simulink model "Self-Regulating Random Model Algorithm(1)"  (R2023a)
settings: Solver=VariableStepAuto  StartTime=0.0  StopTime=20  RelTol=1e-3
libraries: simulink x63, spspowerguiLib x1
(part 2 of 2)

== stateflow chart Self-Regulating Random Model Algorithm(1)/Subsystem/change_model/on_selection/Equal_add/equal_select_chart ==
  state select_num=equal_select(x) [function]
    (default) -> (junction 31)
    (junction 29) -> (junction 65) : {x=x-1}
    (junction 65) -> (junction 118) : [x==0]
    (junction 31) -> (junction 29) : [oo1==1]
    (junction 65) -> (junction 137)
    (junction 118) -> (junction 93) : {select_num=1}
    (junction 31) -> (junction 137)
    (junction 88) -> (junction 91) : {x=x-1}
    (junction 91) -> (junction 89) : [x==0]
    (junction 137) -> (junction 88) : [oo2==1]
    (junction 91) -> (junction 119)
    (junction 89) -> (junction 34) : {select_num=2}
    (junction 137) -> (junction 119)
    (junction 138) -> (junction 142) : {x=x-1}
    (junction 142) -> (junction 143) : [x==0]
    (junction 119) -> (junction 138) : [oo3==1]
    (junction 142) -> (junction 154)
    (junction 143) -> (junction 104) : {select_num=3}
    (junction 119) -> (junction 154)
    (junction 149) -> (junction 153) : {x=x-1}
    (junction 153) -> (junction 155) : [x==0]
    (junction 154) -> (junction 149) : [oo4==1]
    (junction 153) -> (junction 134)
    (junction 155) -> (junction 99) : {select_num=4}
    (junction 154) -> (junction 134)
    (junction 132) -> (junction 131) : {x=x-1}
    (junction 131) -> (junction 128) : [x==0]
    (junction 134) -> (junction 132) : [oo5==1]
    (junction 131) -> (junction 62)
    (junction 128) -> (junction 157) : {select_num=5}
    (junction 134) -> (junction 62)
    (junction 63) -> (junction 61) : {x=x-1}
    (junction 61) -> (junction 59) : [x==0]
    (junction 62) -> (junction 63) : [oo6==1]
    (junction 61) -> (junction 48)
    (junction 59) -> (junction 45) : {select_num=6}
    (junction 62) -> (junction 48)
    (junction 47) -> (junction 46) : {x=x-1}
    (junction 46) -> (junction 49) : [x==0]
    (junction 48) -> (junction 47) : [oo7==1]
    (junction 46) -> (junction 43)
    (junction 49) -> (junction 44) : {select_num=7}
    (junction 48) -> (junction 43)
    (junction 43) -> (junction 35) : [oo8==1]
    (junction 35) -> (junction 41) : {x=x-1}
    (junction 41) -> (junction 39) : [x==0]
    (junction 41) -> (junction 112)
    (junction 43) -> (junction 112)
    (junction 39) -> (junction 148) : {select_num=8}
    (junction 112) -> (junction 111) : [oo9==1]
    (junction 111) -> (junction 110) : {x=x-1}
    (junction 110) -> (junction 107) : [x==0]
    (junction 110) -> (junction 70)
    (junction 112) -> (junction 70)
    (junction 107) -> (junction 95) : {select_num=9}
    (junction 70) -> (junction 69) : [oo10==1]
    (junction 69) -> (junction 67) : {x=x-1}
    (junction 67) -> (junction 66) : [x==0]
    (junction 67) -> (junction 82)
    (junction 70) -> (junction 82)
    (junction 66) -> (junction 122) : {select_num=10}
    (junction 82) -> (junction 86) : [oo11==1]
    (junction 86) -> (junction 79) : {x=x-1}
    (junction 79) -> (junction 84) : [x==0]
    (junction 79) -> (junction 145)
    (junction 82) -> (junction 145)
    (junction 84) -> (junction 96) : {select_num=11}
    (junction 145) -> (junction 102) : {select_num=12}
    (junction 96) -> (junction 102)
    (junction 122) -> (junction 96)
    (junction 95) -> (junction 122)
    (junction 93) -> (junction 34)
    (junction 148) -> (junction 95)
    (junction 45) -> (junction 44)
    (junction 157) -> (junction 45)
    (junction 44) -> (junction 148)
    (junction 102) -> (junction 78)
    (junction 99) -> (junction 157)
    (junction 104) -> (junction 99)
    (junction 34) -> (junction 104)
  state equal_add_select_block
    exit:
  (default) -> equal_add_select_block : {euqal_check_width = 1/Off_num; equal_step=ceil(Random_num/euqal_check_width); Equal_add_num=equal_select(equal_step)}
  equal_add_select_block -> equal_add_select_block : {euqal_check_width = 1/Off_num; equal_step=ceil(Random_num/euqal_check_width); Equal_add_num=equal_select(equal_step)}
  data: select_num function_output double; x function_input double; Off_num input; Random_num input; Equal_add_num output single; oo1 input; oo2 input; oo3 input; oo4 input; oo5 input; oo6 input; oo7 input; oo8 input; oo9 input; oo10 input; oo11 input; oo12 input; euqal_check_width local single; equal_step local single

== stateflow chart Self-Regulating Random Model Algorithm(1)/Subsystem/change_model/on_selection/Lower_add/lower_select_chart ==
  state select_num=lower_select(x) [function]
    (default) -> (junction 28)
    (junction 26) -> (junction 62) : {x=x-1}
    (junction 62) -> (junction 115) : [x==0]
    (junction 28) -> (junction 26) : [oo1==1]
    (junction 62) -> (junction 134)
    (junction 115) -> (junction 90) : {select_num=1}
    (junction 28) -> (junction 134)
    (junction 85) -> (junction 88) : {x=x-1}
    (junction 88) -> (junction 86) : [x==0]
    (junction 134) -> (junction 85) : [oo2==1]
    (junction 88) -> (junction 151)
    (junction 86) -> (junction 31) : {select_num=2}
    (junction 134) -> (junction 151)
    (junction 146) -> (junction 150) : {x=x-1}
    (junction 150) -> (junction 152) : [x==0]
    (junction 151) -> (junction 146) : [oo3==1]
    (junction 150) -> (junction 131)
    (junction 152) -> (junction 96) : {select_num=3}
    (junction 151) -> (junction 131)
    (junction 129) -> (junction 128) : {x=x-1}
    (junction 128) -> (junction 125) : [x==0]
    (junction 131) -> (junction 129) : [oo7==1]
    (junction 128) -> (junction 59)
    (junction 125) -> (junction 154) : {select_num=7}
    (junction 131) -> (junction 59)
    (junction 59) -> (junction 40)
    (junction 40) -> (junction 32) : [oo8==1]
    (junction 32) -> (junction 38) : {x=x-1}
    (junction 38) -> (junction 36) : [x==0]
    (junction 38) -> (junction 109)
    (junction 40) -> (junction 109)
    (junction 36) -> (junction 145) : {select_num=8}
    (junction 109) -> (junction 108) : [oo9==1]
    (junction 108) -> (junction 107) : {x=x-1}
    (junction 107) -> (junction 104) : [x==0]
    (junction 107) -> (junction 67)
    (junction 104) -> (junction 92) : {select_num=9}
    (junction 109) -> (junction 67)
    (junction 67) -> (junction 66) : [oo10==1]
    (junction 66) -> (junction 64) : {x=x-1}
    (junction 64) -> (junction 63) : [x==0]
    (junction 64) -> (junction 142)
    (junction 67) -> (junction 142)
    (junction 63) -> (junction 119) : {select_num=10}
    (junction 142) -> (junction 99) : {select_num=12}
    (junction 119) -> (junction 99)
    (junction 92) -> (junction 119)
    (junction 90) -> (junction 31)
    (junction 145) -> (junction 92)
    (junction 42) -> (junction 145)
    (junction 154) -> (junction 42)
    (junction 31) -> (junction 96)
    (junction 99) -> (junction 75)
    (junction 96) -> (junction 154)
  state lower_add_select_block
    exit:
  (default) -> lower_add_select_block : {lower_check_width = 1/Off_num; lower_step=ceil(Random_num/lower_check_width); Lower_add_num=lower_select(lower_step);}
  lower_add_select_block -> lower_add_select_block : {lower_check_width = 1/Off_num; lower_step=ceil(Random_num/lower_check_width); Lower_add_num=lower_select(lower_step)}
  data: select_num function_output single; x function_input double; Off_num input; Random_num input; Lower_add_num output single; oo1 input; oo2 input; oo3 input; oo7 input; oo8 input; oo9 input; oo10 input; oo12 input; lower_check_width local single; lower_step local single
